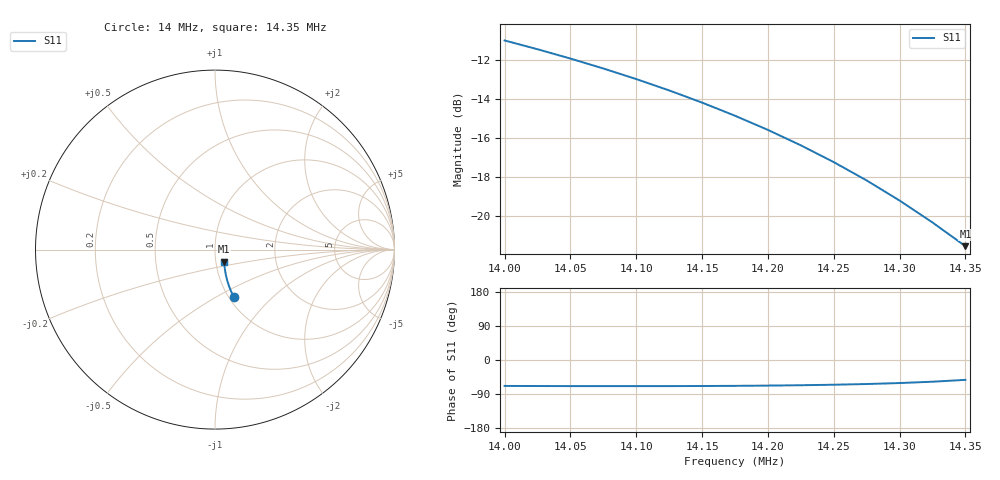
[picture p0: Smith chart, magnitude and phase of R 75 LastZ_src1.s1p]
! EZNEC Pro/4 beta ver. A6.0
! 5/17/2015 1:33:49 PM
! Back yard dipole
! Source 1
# MHZ S MA R 75
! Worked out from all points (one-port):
!   15 points, 14 MHz to 14.35 MHz, reference 75 ohm
!   lowest |S11| = -21.5 dB at 14.35 MHz (marker M1), VSWR 1.18, Z = 82.3 - j11 ohm
!   |S11| at or under -10 dB: start of sweep to end of sweep
14  0.2818 -68.4
14.025  0.2676 -68.7
14.05  0.2533 -68.9
14.075  0.2389 -69.0
14.1  0.2244 -69.0
14.125  0.2099 -68.9
14.15  0.1953 -68.6
14.175  0.1808 -68.2
14.2  0.1663 -67.6
14.225  0.1518 -66.6
14.25  0.1375 -65.2
14.275  0.1234 -63.4
14.3  0.1096 -60.8
14.325  0.09633 -57.3
14.35  0.08376 -52.4
